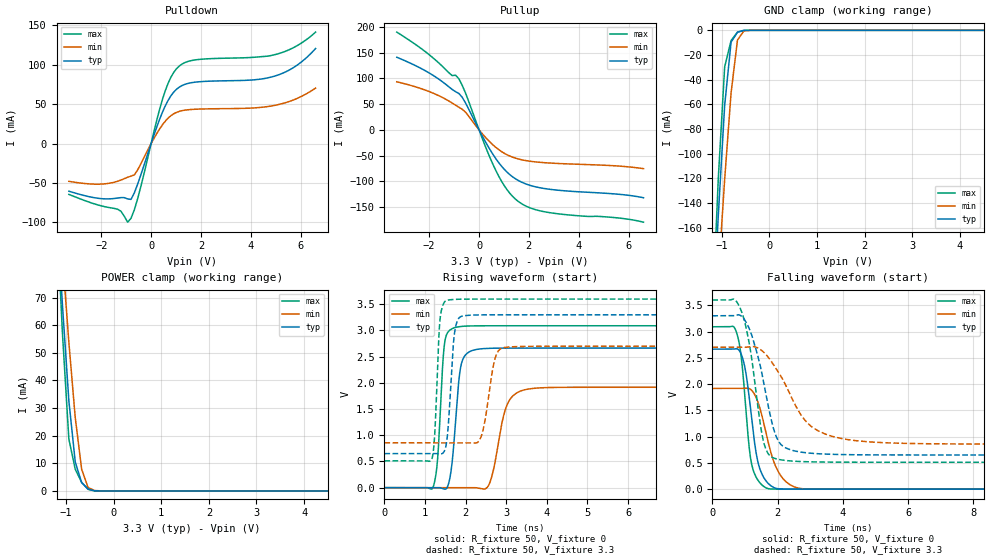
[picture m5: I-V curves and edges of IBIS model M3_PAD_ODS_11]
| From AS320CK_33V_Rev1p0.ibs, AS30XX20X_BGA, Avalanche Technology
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[Model] M3_PAD_ODS_11
Model_type I/O
Enable   Active-High
Vinl  =  0.8
Vinh  =  2.2
Vmeas =  1.65
Cref  =  30e-12
| Capacitance  typ   min   max
C_comp   1.518728e-12   1.426995e-12   1.652439e-12
| Variables   typ   min   max
[GND Clamp Reference]   0   0   0
[POWER Clamp Reference]   3.3   2.7   3.6
[Pulldown Reference]   0   0   0
[Pullup Reference]   3.3   2.7   3.6
[Temperature Range]   25   125   -40
[Voltage Range]   3.3   2.7   3.6
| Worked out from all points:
|   slope of the pulldown table from 0 to 0.495 V, typ, clamps not added: 11.6 ohm
|   slope of the pullup table from 0 to 0.495 V, typ, clamps not added: 11.6 ohm
|   GND clamp passes 1 mA (typ) near -0.62 V on its own axis
|   POWER clamp passes 1 mA (typ) near -0.56 V on its own axis
|   falling waveform, R_fixture 50, V_fixture 0: 20-80 % time 343ps typ, 517ps min, 271ps max; typ from 2.67 V to 0 V
|   falling waveform, R_fixture 50, V_fixture 3.3: 20-80 % time 577ps typ, 1.06ns min, 431ps max; typ from 3.3 V to 0.65 V
|   rising waveform, R_fixture 50, V_fixture 0: 20-80 % time 171ps typ, 299ps min, 130ps max; typ from 0 V to 2.67 V
|   rising waveform, R_fixture 50, V_fixture 3.3: 20-80 % time 129ps typ, 221ps min, 101ps max; typ from 0.65 V to 3.3 V
[GND Clamp]
| Voltage   I(typ)   I(min)   I(max)
-3.3V     -1.961A    -1.697A    -2.357A
-1.21V    -250.6mA   -283.7mA   -242.3mA
-1.076V   -150.5mA   -200.1mA   -120.5mA
-941.4mV  -60.74mA   -120.8mA   -29.57mA
-806.9mV  -9.575mA   -50.7mA    -8.297mA
-672.4mV  -1.554mA   -7.862mA   -1.403mA
-537.9mV  -68.54uA   -503.1uA   -16.86uA
-403.4mV  -562.8nA   -18.5uA    -33.35nA
6.6V      0A         0A         0A
[POWER Clamp]
| Voltage   I(typ)   I(min)   I(max)
-3.3V     772.3mA    673.3mA    930.5mA
-1.21V    105.9mA    117.6mA    104.6mA
-1.076V   67.34mA    85.06mA    57.16mA
-941.4mV  32.71mA    53.93mA    18.82mA
-806.9mV  10.48mA    26.53mA    7.848mA
-672.4mV  2.975mA    7.856mA    3.108mA
-537.9mV  710.9uA    1.248mA    573.1uA
-403.4mV  60.69uA    160.8uA    9.187uA
-269mV    142.4nA    6.118uA    23.26nA
6.6V      0A         0A         0A
[Pulldown]
| Voltage   I(typ)   I(min)   I(max)
-3.3V     -60.37mA   -47.84mA   -64.43mA
-1.345V   -69.07mA   -47.77mA   -83.25mA
-941.4mV  -70.2mA    -42.7mA    -99.71mA
-806.9mV  -70.75mA   -41.25mA   -94.81mA
-537.9mV  -51.24mA   -33.31mA   -69.65mA
455.2mV   39.84mA    23.83mA    56.08mA
682.8mV   54.89mA    32.35mA    76.58mA
1.024V    69.09mA    39.7mA     95.16mA
1.821V    78.16mA    43.68mA    106.4mA
4.914V    85.23mA    48.22mA    112.5mA
5.783V    97.9mA     56.32mA    122.9mA
6.6V      120.6mA    70.51mA    141.5mA
[Pullup]
| Voltage   I(typ)   I(min)   I(max)
-3.3V     140.8mA    93.23mA    189.7mA
-1.883V   106.9mA    71.94mA    141.1mA
-1.076V   78.23mA    51.91mA    105.2mA
-941.4mV  74mA       47.77mA    106.1mA
-806.9mV  70.44mA    43.77mA    98.95mA
-537.9mV  51.81mA    33.92mA    70.93mA
227.6mV   -20.69mA   -13mA      -28.86mA
682.8mV   -56.63mA   -34.49mA   -79.79mA
1.138V    -82.79mA   -48.78mA   -117.2mA
1.593V    -98.83mA   -56.79mA   -139.7mA
2.731V    -114.8mA   -64.18mA   -160mA
6.6V      -131.9mA   -75.47mA   -179.4mA
[Ramp]
dV/dt_r   1.59883/0.171259n  1.15002/0.298673n  1.85445/0.129635n
dV/dt_f   1.58992/0.576881n  1.10595/1.05784n  1.85299/0.431495n
R_load = 50
[Falling Waveform]
R_fixture = 50
V_fixture = 0
V_fixture_min = 0
V_fixture_max = 0
| Time   V(typ)   V(min)   V(max)
0s        2.665V     1.917V     3.091V
741.5ps   2.672V     1.917V     2.983V
875.1ps   2.582V     1.917V     2.564V
986.9ps   2.346V     1.919V     1.835V
1.188ns   1.432V     1.891V     524.1mV
1.408ns   488.3mV    1.639V     160.7mV
1.706ns   112.7mV    908.9mV    10.33mV
2.112ns   2.837mV    241.9mV    1.391mV
2.791ns   846.1uV    6.35mV     485.7uV
21.88ns   -115.7nV   -19.39nV   -933.8nV
[Falling Waveform]
R_fixture = 50
V_fixture = 3.3
V_fixture_min = 2.7
V_fixture_max = 3.6
| Time   V(typ)   V(min)   V(max)
0s        3.3V       2.7V       3.6V
660.8ps   3.301V     2.7V       3.617V
882.6ps   3.297V     2.701V     3.4V
1.153ns   3.022V     2.713V     2.693V
1.559ns   2.075V     2.615V     929.2mV
1.718ns   1.565V     2.508V     668mV
2.009ns   934.3mV    2.24V      569.3mV
2.973ns   686.3mV    1.224V     520.4mV
4.385ns   655mV      923.6mV    512.5mV
21.88ns   650.1mV    856.7mV    511.7mV
[Rising Waveform]
R_fixture = 50
V_fixture = 0
V_fixture_min = 0
V_fixture_max = 0
| Time   V(typ)   V(min)   V(max)
0s        4.704nV    37.51nV    -841.1pV
1.193ns   846.3uV    522.7uV    1.11mV
1.308ns   928.3uV    573.4uV    538.4mV
1.48ns    -26.9mV    648.6uV    2.751V
1.64ns    311.9mV    718.5uV    3.023V
1.798ns   1.752V     787.9uV    3.067V
2.543ns   2.658V     17.22mV    3.09V
3.03ns    2.664V     1.597V     3.091V
3.603ns   2.665V     1.889V     3.091V
21.88ns   2.665V     1.917V     3.091V
[Rising Waveform]
R_fixture = 50
V_fixture = 3.3
V_fixture_min = 2.7
V_fixture_max = 3.6
| Time   V(typ)   V(min)   V(max)
0s        650.1mV    856.8mV    511.7mV
1.167ns   651mV      856.4mV    547.5mV
1.368ns   647.9mV    856.4mV    3.202V
1.576ns   1.226V     856.3mV    3.582V
1.735ns   3V         856.2mV    3.594V
1.976ns   3.283V     856.2mV    3.599V
2.366ns   3.298V     942.7mV    3.6V
2.719ns   3.299V     2.451V     3.6V
3.001ns   3.299V     2.68V      3.6V
21.88ns   3.3V       2.7V       3.6V
